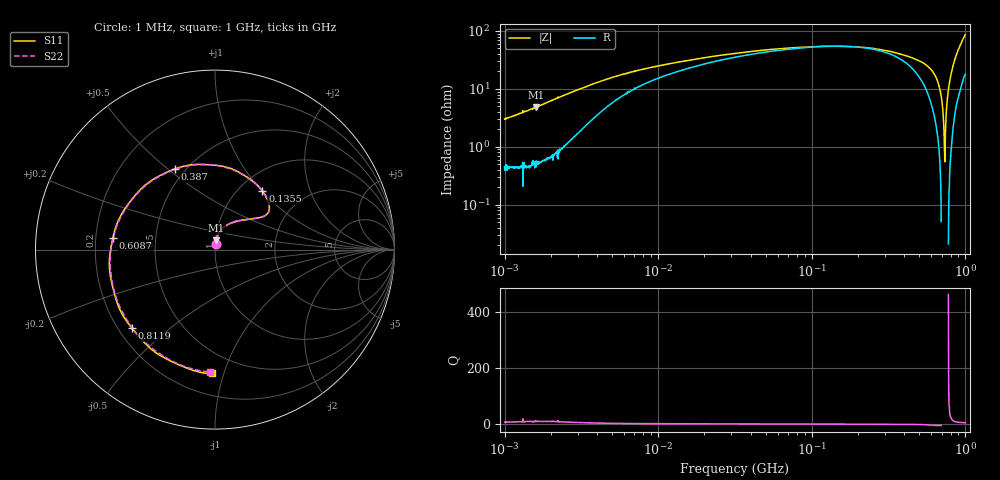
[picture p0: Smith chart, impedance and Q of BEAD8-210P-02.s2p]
!s-Parameter Generated by FASTRON Sdn. Bhd.
!FASTRON P/N : BEAD/8-210P
!Vector Network Analyser E5071C,MY46733604,B.14.02
!Date: Mon Jul 31 13:15:55 2023
!Data & Calibration Information:
!Freq	S11:SOLT2(ON)	S21:SOLT2(ON)	S12:SOLT2(ON)	S22:SOLT2(ON)
!PortZ  Port1:50+j0  Port2:50+j0
!When reading, reference impedance value at option line is always used.
! Remarks : This data is being provided solely for informational purposes.
# Hz S dB R 50
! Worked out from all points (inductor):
!   1601 points, 1 MHz to 1 GHz, reference 50 ohm
!   read as one part in series: L = 473 nH near 1.041 MHz
!   highest Q = 9.65 at 1.601 MHz (marker M1), where L = 481 nH
!   self-resonance near 162.7 MHz
!   S11 on the Smith chart (normalised r, x): 1 MHz: 1.01, +0.07; 135.5 MHz: 1.27, +1.01; 387 MHz: 0.44, +0.53; 608.7 MHz: 0.27, +0.05; 811.9 MHz: 0.26, -0.38; 1 GHz: 0.35, -0.92
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1000000  -29.62 79.1  -0.03 -1.5  -0.04 -1.6  -29.78 79.1
1600700  -25.69 82.6  -0.04 -2.6  -0.05 -2.6  -25.92 81.3
2203310  -22.69 80.1  -0.07 -3.5  -0.07 -3.6  -22.67 80.9
3167252  -19.48 74.7  -0.23 -5.2  -0.22 -5.2  -19.50 74.6
5180540  -15.91 62.0  -0.62 -7.4  -0.62 -7.4  -15.90 62.0
1.002882e7  -12.91 46.6  -1.39 -8.3  -1.40 -8.3  -12.87 46.5
3.163788e7  -9.72 34.4  -2.81 -3.9  -2.81 -3.9  -9.71 34.5
5.725233e7  -8.67 35.6  -3.48 2.5  -3.47 2.5  -8.67 35.4
1.00144e8  -7.92 43.0  -4.00 12.8  -4.00 12.8  -7.92 43.0
1.354532e8  -7.52 51.0  -4.25 21.0  -4.24 21.0  -7.55 51.0
2.156097e8  -6.96 71.1  -4.59 39.0  -4.59 39.0  -6.98 71.3
3.171813e8  -6.40 97.9  -4.88 61.1  -4.87 61.1  -6.40 97.8
3.870464e8  -5.99 116.4  -5.04 76.0  -5.04 76.1  -6.02 116.1
4.386022e8  -5.71 129.5  -5.19 87.1  -5.19 87.2  -5.75 129.6
4.90158e8  -5.43 143.2  -5.31 98.0  -5.30 98.1  -5.47 142.9
5.422962e8  -5.16 156.2  -5.46 109.2  -5.46 109.2  -5.22 156.2
6.087073e8  -4.85 173.3  -5.63 123.2  -5.64 123.3  -4.88 173.1
7.043391e8  -4.38 -162.8  -5.92 143.4  -5.92 143.6  -4.44 -163.0
7.602749e8  -4.09 -149.1  -6.10 155.5  -6.10 155.5  -4.17 -149.2
8.11908e8  -3.92 -136.5  -6.27 166.2  -6.28 166.3  -3.95 -136.7
9.004219e8  -3.53 -115.0  -6.59 -175.2  -6.60 -175.1  -3.61 -115.5
1e9  -3.23 -91.2  -7.09 -154.4  -7.08 -154.2  -3.32 -92.2
